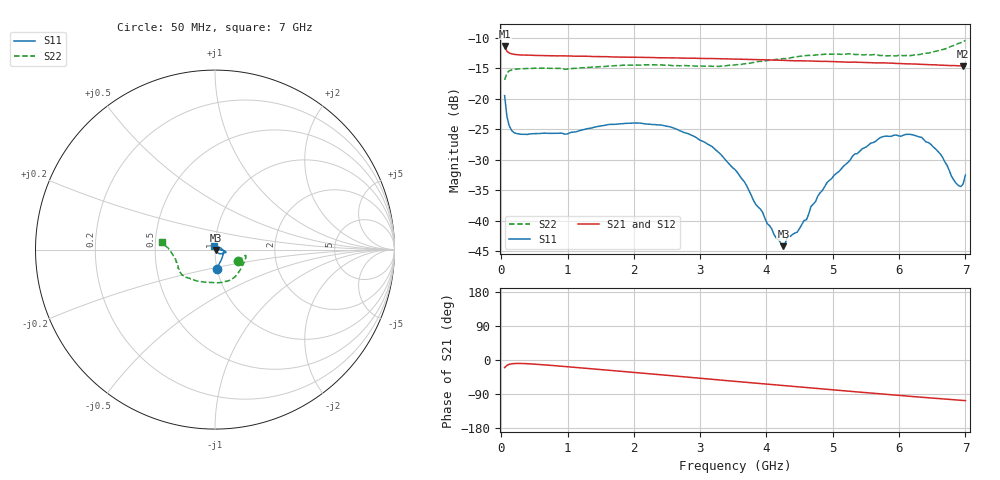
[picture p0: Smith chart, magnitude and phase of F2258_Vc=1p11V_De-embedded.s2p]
! Integrated Device Technology
! Corporate Headquarters
! 6024 Silver Creek Valley Road
! San Jose, CA 95138  USA
! Phone:  1-408-284-8200
! Toll Free:  1-800-223-1366
! Webpage:  http://www.idt.com/
! Timing and RF Division
! 515 Groton Road, Suite 102
! Westford, MA 01886-6024
! Device:  F2258
! Description: Voltage Variable RF Attenuator
! Frequency:  50.0 -  6000.00 MHz
! Package:  3x3 mm Thin QFN Plastic Package: 16 pin
! Ports:  2 RF, 2 DC
!  Pin  1  = NC
!  Pin  2  = NC
!  Pin  3  = RF2  = Port 2
!  Pin  4  = GND
!  Pin  5  = Vdd
!  Pin  6  = NC
!  Pin  7  = VCTRL
!  Pin  8  = NC
!  Pin  9  = GND
!  Pin 10  = RF1  = Port 1
!  Pin 11  = NC
!  Pin 12  = NC
!  Pin 13  = NC
!  Pin 14  = NC
!  Pin 15  = NC
!  Pin 16  = NC
! Vcntrl:  1.110 Volts
! Vdd:  +3.300 Volts
! Current:  1.165 mA
! Data:  The device was measured on a the F2258 evaluation board which has
!  individual transmission lines to the RF pins.  Data was collected
!  using a calibrated network analyzer.  The evaluation board was
!  de-embedded using a TRL calibration technique.
!  The reference plane is the edge of the package pin.
! Misc:  SN 10
!  Action Tracker AT0285
! Date Measured:  2014-12-10
! Date:  2016-01-13  MJV
! Note:
!  Integrated Device Technology supplies this data as a sample of measured
!  data at the package pin for this product.  Your particular data for this
!  product may vary.
!  Data was taken at 25 degrees C.
!  Integrated Device Technology reserves the right to change this data at anytime.
!Freq_(GHz)  S11M_(dB)  S11P_(deg)  S21M_(dB)  S21P_(deg)  S12M_(dB)  S12P_(deg)  S22M_(dB)  S22P_(deg)
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# GHz S dB R 50
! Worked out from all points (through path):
!   201 points, 50 MHz to 7 GHz, reference 50 ohm
!   highest |S21| = -11.35 dB at 50 MHz (marker M1); lowest = -14.7 dB at 6.965 GHz (marker M2)
!   group delay of S21, straight-line fit = 41.3 ps
!   lowest |S11| = -44.2 dB at 4.255 GHz (marker M3), VSWR 1.01, Z = 50.5 - j0.417 ohm
!   |S11| at or under -10 dB: start of sweep to end of sweep
!   |S22| runs from -16.9 to -10.5 dB; largest |S21 - S12| = 0.0013
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0.05  -19.50 -85.1  -11.35 -20.0  -11.34 -19.9  -16.93 -26.7
0.08475  -22.92 -63.6  -12.22 -14.2  -12.21 -14.2  -15.80 -14.9
0.1195  -24.44 -48.8  -12.51 -11.5  -12.52 -11.5  -15.42 -12.0
0.189  -25.55 -33.1  -12.73 -9.5  -12.73 -9.5  -15.21 -10.8
0.98825  -25.81 -18.5  -12.99 -17.6  -12.99 -17.6  -15.16 -31.0
1.2315  -25.10 -17.3  -13.05 -21.2  -13.04 -21.2  -14.91 -37.4
2.37825  -24.31 -10.3  -13.29 -38.5  -13.26 -38.5  -14.46 -66.5
3.1775  -27.84 -4.5  -13.42 -51.0  -13.44 -50.9  -14.69 -92.3
3.525  -31.63 -3.0  -13.50 -56.4  -13.53 -56.4  -14.47 -106.1
4.25475  -44.19 -42.0  -13.72 -67.7  -13.75 -67.6  -13.42 -129.9
4.32425  -42.58 -50.2  -13.75 -68.8  -13.78 -68.7  -13.41 -131.7
4.46325  -41.88 -63.4  -13.78 -70.9  -13.81 -70.9  -13.12 -135.4
4.60225  -39.85 -64.2  -13.81 -72.9  -13.84 -72.9  -12.92 -137.8
4.7065  -37.28 -59.2  -13.84 -74.5  -13.88 -74.5  -12.89 -139.6
4.915  -33.72 -53.9  -13.89 -77.6  -13.94 -77.6  -12.72 -142.7
5.332  -29.06 -39.2  -14.00 -83.8  -14.05 -83.7  -12.76 -148.8
5.85325  -26.18 -23.8  -14.17 -91.3  -14.20 -91.3  -12.95 -158.6
6.33975  -26.32 -8.3  -14.37 -98.3  -14.41 -98.3  -12.69 -170.7
6.61775  -29.03 11.7  -14.50 -102.1  -14.51 -102.1  -12.07 -178.5
6.861  -33.89 55.4  -14.59 -105.5  -14.64 -105.4  -11.12 175.4
6.96525  -34.02 94.2  -14.66 -106.9  -14.69 -106.7  -10.66 173.1
7  -32.54 105.9  -14.66 -107.2  -14.70 -107.2  -10.45 172.2
